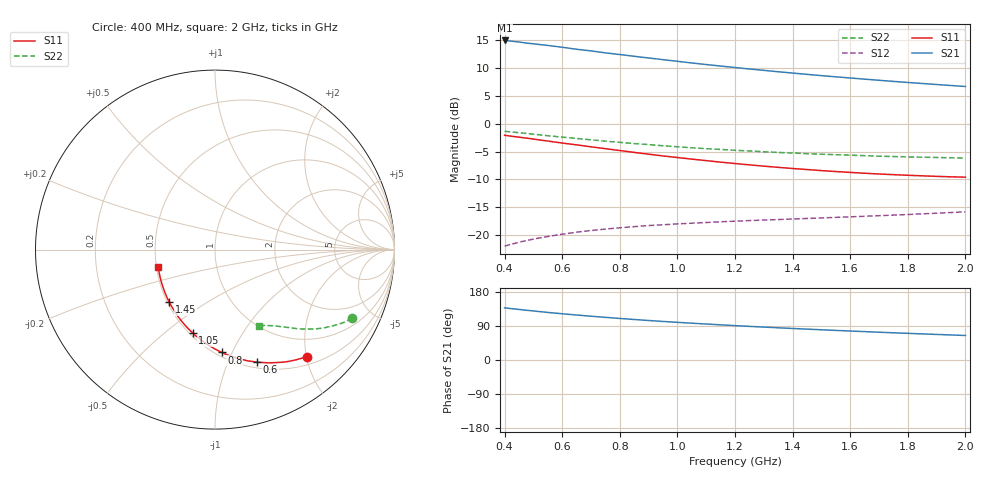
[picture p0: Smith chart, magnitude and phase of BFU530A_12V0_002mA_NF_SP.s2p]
! Filename:  P:\Prog\Test\Noise\ATS_data\Testdata_Net\06 Compressed Noise after Statistics\BFU530A_APG2013_33_A05_12p0V_002mA_NF_CM01_D.sf
! Date/Time: Tue 16/Apr/2013 15:11:00
! BFU530A_APG2013_33_A05_12p0V_1to25mA_NF_CM01_Bias2_R.sf
! Noise Parameter Data File
! BFU530A_APG2013_33_A05_12p0V_1to25mA_NF_CM01
! Date/time: Fri Apr 12 17:55:00 2013
! VAR V_out= 12.001000
! VAR I_out= 1.990000
! VAR V_in= 0.793100
! VAR I_in= 0.015800
! Device data file deembeded for feedlines and parallel
! Original file: \06 Compressed Noise after Statistics\BFU530A_APG2013_33_A05_12p0V_002mA_NF_CM01_R.sf
! Feed-files: PR017V01_150413_Feed1.s2p, PR017V01_150413_Feed2.s2p
! Parallel-file: PR017V01_150413_Par.s2p
# MHz S MA R 50
!  Freq-MHz  S11-mag  S11-arg  S21-mag  S21-arg  S12-mag  S12-arg  S22-mag  S22-arg
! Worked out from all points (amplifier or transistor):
!   37 points, 400 MHz to 2 GHz, reference 50 ohm
!   highest |S21| = 14.9 dB at 400 MHz (marker M1)
!   |S21| within 3 dB of that: start of sweep to 875.9 MHz
!   unconditionally stable (mu >= 1): nowhere
!   at 500 MHz: K = 0.33, MSG = 17.5 dB, |S12| = -20.7 dB
!   at 1.1 GHz: K = 0.67, MSG = 14.2 dB, |S12| = -17.7 dB
!   at 2 GHz: K = 0.99, MSG = 11.3 dB, |S12| = -15.8 dB
!   lowest NFmin = 0.52 dB at 420 MHz
!   S11 on the Smith chart (normalised r, x): 400 MHz: 0.65, -2.01; 600 MHz: 0.56, -1.28; 800 MHz: 0.53, -0.91; 1.05 GHz: 0.52, -0.63; 1.45 GHz: 0.51, -0.35; 2 GHz: 0.51, -0.11
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400  0.786 -49.3  5.582 137.6  0.07952 62.1  0.8538 -26.6
420  0.7739 -51.5  5.517 135.8  0.08232 61.1  0.8439 -27.6
440  0.7626 -53.6  5.441 134.2  0.08494 60.2  0.8342 -28.5
500  0.7272 -59.8  5.211 129.4  0.09212 57.5  0.8045 -31.1
550  0.6979 -64.7  5.035 125.5  0.09714 55.6  0.7793 -33.1
600  0.67 -69.4  4.852 122.0  0.1018 54.0  0.7569 -34.9
650  0.6455 -73.7  4.653 118.8  0.1062 52.5  0.7367 -36.5
700  0.6193 -78.2  4.498 115.5  0.1098 51.2  0.716 -38.0
750  0.5965 -82.2  4.319 112.5  0.1132 50.1  0.6973 -39.4
800  0.5739 -86.4  4.173 109.7  0.1163 49.1  0.6796 -40.6
850  0.5521 -90.4  4.024 106.9  0.1191 48.2  0.663 -41.8
900  0.532 -94.2  3.886 104.2  0.1218 47.5  0.6491 -42.9
950  0.5134 -97.9  3.755 101.8  0.1238 47.0  0.6332 -44.0
1050  0.4805 -105.1  3.506 97.1  0.1278 46.2  0.6074 -45.8
1100  0.4658 -108.5  3.394 94.9  0.1297 45.9  0.5963 -46.7
1200  0.4387 -115.3  3.191 90.8  0.1332 45.5  0.5768 -48.3
1300  0.4156 -121.8  3.01 86.8  0.1364 45.5  0.5601 -49.9
1450  0.3875 -131.3  2.771 81.5  0.1409 46.0  0.5381 -52.1
1500  0.3791 -134.4  2.698 79.7  0.1425 46.2  0.532 -52.8
1650  0.3589 -143.3  2.509 74.9  0.1475 47.2  0.5163 -55.0
1750  0.3486 -149.2  2.395 71.8  0.1511 48.2  0.507 -56.4
2000  0.331 -163.0  2.157 64.7  0.1617 50.5  0.4914 -60.1
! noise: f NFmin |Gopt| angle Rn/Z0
400  0.5828  0.4677  21.5  0.2085
460  0.5864  0.4567  28.51  0.1981
600  0.6539  0.4656  30.85  0.2098
800  0.6605  0.4234  50.15  0.1677
1000  0.7098  0.4185  62.2  0.1532
1200  0.7543  0.4076  75.32  0.1482
1400  0.7803  0.3904  90.56  0.1251
1600  0.8366  0.3989  108.2  0.0951
1800  0.82  0.3759  118.2  0.0871
2000  0.8216  0.3847  137.9  0.0693
